(* Logix 5000 AddOnInstructionDefinition export Banner_Q5X_PD_v4; software revision 33.00 *)

TYPE Banner_Q5X_PD0_v4 :   // Process Data 0 for a Q5X 2000, 3000, or 5000.
STRUCT
   C1_Output_State : SINT;   // 0 = Inactive, 1 = Active
   C2_Output_State : SINT;   // 0 = Inactive, 1 = Active
   Stability : SINT;   // 0 = No target or Marginal, 1 = Stable
   Measurement_1 : DINT;
   Measurement_2 : DINT;
END_STRUCT
END_TYPE

TYPE Banner_Q5X_PD1_v4 :   // Process Data 1 for a Q5X 2000, 3000, or 5000.
STRUCT
   Measurement_1 : DINT;
   Measurement_2 : DINT;
END_STRUCT
END_TYPE

TYPE Banner_Q5X_PD2_v4 :   // Process Data 2 for a Q5X 2000, 3000, or 5000.
STRUCT
   Measurement : DINT;   // Measurement Value
   Measure_Scale : DINT;   // Scale Factor for Measurement
   Stability : SINT;   // 0 = Inactive 1 = Active
   Channel_1 : SINT;   // 0 = Inactive 1 = Active
   Channel_2 : INT;   // 0 = Inactive 1 = Active
END_STRUCT
END_TYPE

TYPE Banner_Q5X_PDIO_v4 :   // Process Data for a Q5X 2000, 3000, or 5000
STRUCT
   PDI_0 : Banner_Q5X_PD0_v4;   // Input Procoess Data for Configuration 0
   PDI_1 : Banner_Q5X_PD1_v4;   // Input Procoess Data for Configuration 1
   PDI_2 : Banner_Q5X_PD2_v4;   // Input Procoess Data for Configuration 2
   Transducer_Disable : SINT;   // 0 = Active 1 = Inactive
   PDI_DT : SINT[4];
END_STRUCT
END_TYPE

ADD_ON_INSTRUCTION Banner_Q5X_PD_v4   (* revision 4.0, vendor Banner Engineering *)
// Take raw process data and convert it to usable values.
VAR_IN_OUT
   PD : Banner_Q5X_PDIO_v4; {required}   // Process Data for a Q5X.
END_VAR
VAR_INPUT
   Configuration : SINT; {required}
   Byte_Swap : BOOL; {required}
END_VAR
VAR
   TempI : SINT[4]; {access None}
END_VAR

ROUTINE Logic   (* ladder *)
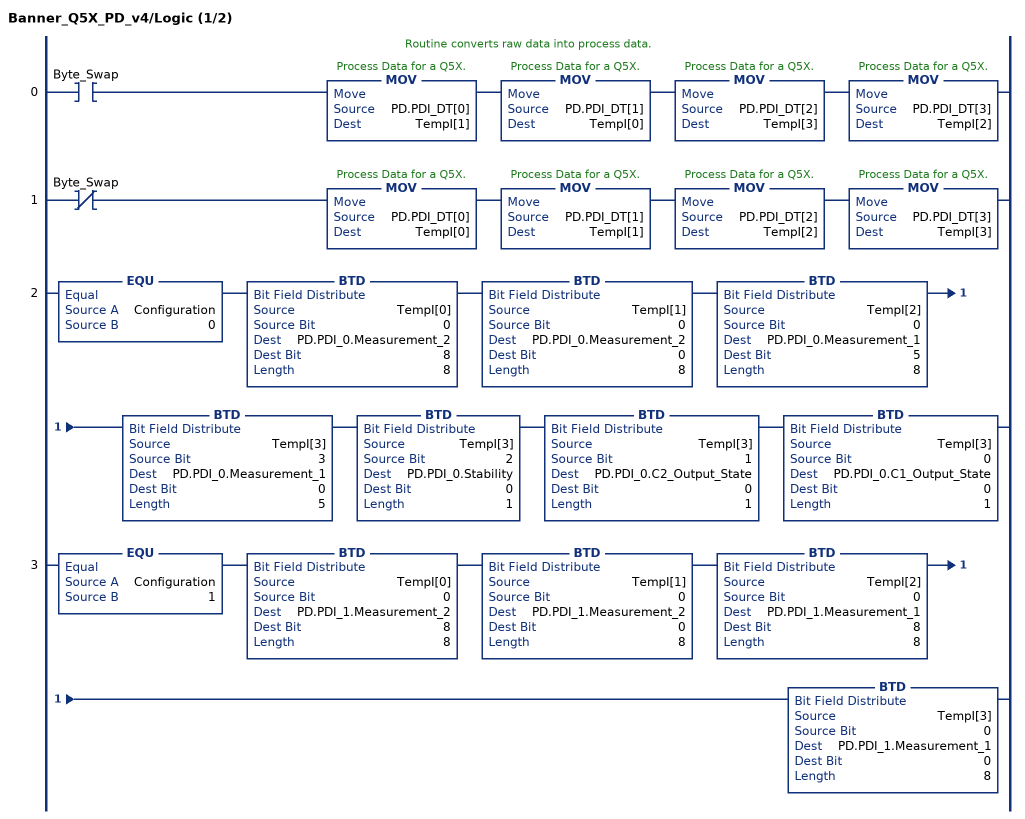
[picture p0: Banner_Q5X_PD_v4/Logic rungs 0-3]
   // Routine converts raw data into process data.
   0: XIC(Byte_Swap)MOV(PD.PDI_DT[0],TempI[1])MOV(PD.PDI_DT[1],TempI[0])MOV(PD.PDI_DT[2],TempI[3])MOV(PD.PDI_DT[3],TempI[2]);
   1: XIO(Byte_Swap)MOV(PD.PDI_DT[0],TempI[0])MOV(PD.PDI_DT[1],TempI[1])MOV(PD.PDI_DT[2],TempI[2])MOV(PD.PDI_DT[3],TempI[3]);
   2: EQU(Configuration,0)BTD(TempI[0],0,PD.PDI_0.Measurement_2,8,8)BTD(TempI[1],0,PD.PDI_0.Measurement_2,0,8)BTD(TempI[2],0,PD.PDI_0.Measurement_1,5,8)BTD(TempI[3],3,PD.PDI_0.Measurement_1,0,5)BTD(TempI[3],2,PD.PDI_0.Stability,0,1)BTD(TempI[3],1,PD.PDI_0.C2_Output_State,0,1)BTD(TempI[3],0,PD.PDI_0.C1_Output_State,0,1);
   3: EQU(Configuration,1)BTD(TempI[0],0,PD.PDI_1.Measurement_2,8,8)BTD(TempI[1],0,PD.PDI_1.Measurement_2,0,8)BTD(TempI[2],0,PD.PDI_1.Measurement_1,8,8)BTD(TempI[3],0,PD.PDI_1.Measurement_1,0,8);
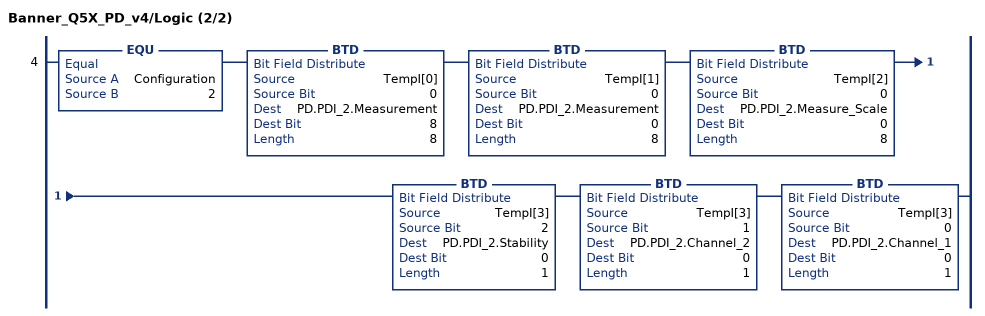
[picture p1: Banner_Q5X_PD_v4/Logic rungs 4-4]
   4: EQU(Configuration,2)BTD(TempI[0],0,PD.PDI_2.Measurement,8,8)BTD(TempI[1],0,PD.PDI_2.Measurement,0,8)BTD(TempI[2],0,PD.PDI_2.Measure_Scale,0,8)BTD(TempI[3],2,PD.PDI_2.Stability,0,1)BTD(TempI[3],1,PD.PDI_2.Channel_2,0,1)BTD(TempI[3],0,PD.PDI_2.Channel_1,0,1);
END_ROUTINE
END_ADD_ON_INSTRUCTION
